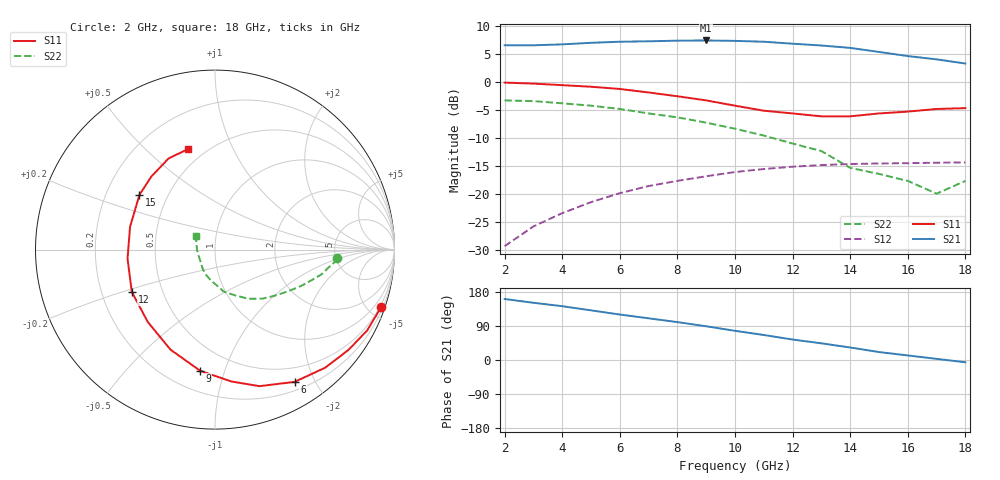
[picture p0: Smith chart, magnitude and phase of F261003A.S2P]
!ATF-26100
!S-PARAMETERS at Vds=3V  Id=10mA.  LAST UPDATED 07-22-92
# ghz s ma r 50
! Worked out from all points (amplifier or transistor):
!   17 points, 2 GHz to 18 GHz, reference 50 ohm
!   highest |S21| = 7.3 dB at 9 GHz (marker M1)
!   |S21| within 3 dB of that: start of sweep to 16.36 GHz
!   unconditionally stable (mu >= 1): 11.98 GHz to end of sweep
!   at 4 GHz: K = 0.43, MSG = 15.1 dB, |S12| = -23.5 dB
!   at 10 GHz: K = 0.89, MSG = 11.7 dB, |S12| = -16.1 dB
!   at 18 GHz: K = 1.32, MAG = 5.4 dB, |S12| = -14.4 dB
!   lowest NFmin = 1.30 dB at 6 GHz
!   S11 on the Smith chart (normalised r, x): 2 GHz: 0.37, -5.95; 6 GHz: 0.31, -1.73; 9 GHz: 0.33, -0.83; 12 GHz: 0.33, -0.21; 15 GHz: 0.35, +0.29; 18 GHz: 0.41, +0.68
2  0.98 -19.0  2.11 161.0  0.034 82.0  0.68 -4.0
3  0.96 -28.0  2.11 151.0  0.051 78.0  0.67 -6.0
4  0.93 -37.0  2.15 142.0  0.067 74.0  0.64 -9.0
5  0.9 -47.0  2.22 131.0  0.084 69.0  0.61 -13.0
6  0.86 -59.0  2.27 120.0  0.101 64.0  0.57 -17.0
7  0.8 -72.0  2.29 110.0  0.117 59.0  0.52 -23.0
8  0.74 -83.0  2.32 100.0  0.13 54.0  0.48 -28.0
9  0.68 -97.0  2.33 89.0  0.143 48.0  0.43 -36.0
10  0.61 -114.0  2.31 77.0  0.156 42.0  0.38 -46.0
11  0.55 -133.0  2.27 66.0  0.166 35.0  0.33 -56.0
12  0.52 -153.0  2.18 54.0  0.174 28.0  0.28 -66.0
13  0.49 -174.0  2.1 44.0  0.18 21.0  0.24 -78.0
14  0.49 165.0  2 33.0  0.184 10.0  0.17 -99.0
15  0.52 144.0  1.84 21.0  0.186 6.0  0.15 -109.0
16  0.54 131.0  1.69 12.0  0.187 3.0  0.13 -121.0
17  0.57 117.0  1.58 3.0  0.189 -6.0  0.1 -177.0
18  0.58 105.0  1.45 -6.0  0.19 -12.0  0.13 145.0
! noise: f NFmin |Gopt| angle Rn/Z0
6  1.3  0.67  52  1.08
8  1.5  0.45  84  1.03
12  1.8  0.22  158  0.84
14  2  0.33  -136  0.91
